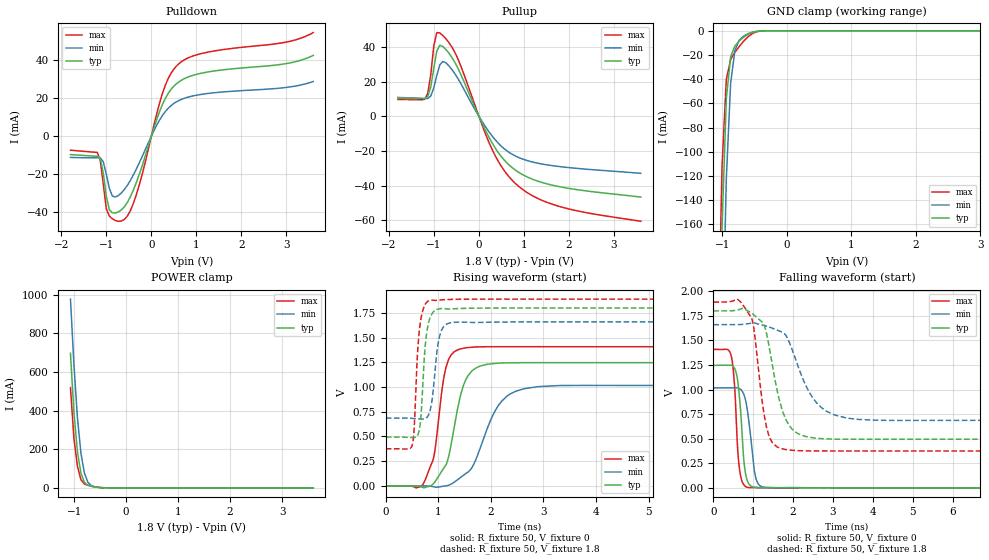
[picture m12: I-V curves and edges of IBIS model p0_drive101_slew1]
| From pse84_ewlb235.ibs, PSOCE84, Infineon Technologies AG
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[Model] p0_drive101_slew1
Model_type I/O
Polarity  Inverting
Enable   Active-High
Vinl  =  0.54
Vinh  =  1.26
Vmeas =  0.9
Cref  =  15pF
| Capacitance   typ   min   max
C_comp   1.253838e-12   1.215159e-12   1.300411e-12
| Variables   typ   min   max
[GND Clamp Reference]   0   0   0
[POWER Clamp Reference]   1.8   1.66   1.89
[Pulldown Reference]   0   0   0
[Pullup Reference]   1.8   1.66   1.89
[Temperature Range]   25   125   -40
[Voltage Range]   1.8   1.66   1.89
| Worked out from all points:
|   slope of the pulldown table from 0 to 0.27 V, typ, clamps not added: 15.1 ohm
|   slope of the pullup table from 0 to 0.27 V, typ, clamps not added: 19 ohm
|   GND clamp passes 1 mA (typ) near -0.51 V on its own axis
|   POWER clamp passes 1 mA (typ) near -0.47 V on its own axis
|   rising waveform, R_fixture 50, V_fixture 0: 20-80 % time 295ps typ, 484ps min, 207ps max; typ from 0 V to 1.25 V
|   rising waveform, R_fixture 50, V_fixture 1.8: 20-80 % time 99.9ps typ, 120ps min, 91.4ps max; typ from 0.495 V to 1.8 V
|   falling waveform, R_fixture 50, V_fixture 0: 20-80 % time 135ps typ, 172ps min, 115ps max; typ from 1.25 V to 0 V
|   falling waveform, R_fixture 50, V_fixture 1.8: 20-80 % time 408ps typ, 637ps min, 275ps max; typ from 1.8 V to 0.495 V
[GND Clamp]
| Voltage   I(typ)   I(min)   I(max)
-1.137V   -619.5mA   -754.2mA   -533mA
-1.07V    -361.2mA   -498.1mA   -281.3mA
-1.003V   -163.8mA   -277.7mA   -113mA
-936.6mV  -56.22mA   -122.3mA   -40.06mA
-869.7mV  -21.33mA   -43.3mA    -23.67mA
-802.8mV  -12.5mA    -15.96mA   -17.71mA
-735.9mV  -8.346mA   -7.675mA   -12.88mA
-669mV    -5.267mA   -4.349mA   -8.575mA
-535.2mV  -1.314mA   -1.207mA   -2.328mA
-401.4mV  -73.55uA   -132.2uA   -119.3uA
3.6V      0A         0A         0A
[POWER Clamp]
| Voltage   I(typ)   I(min)   I(max)
-1.07V    696.7mA    977.2mA    518.8mA
-1.003V   390.1mA    637.2mA    255.1mA
-936.6mV  187.1mA    363.9mA    112.4mA
-869.7mV  77.2mA     180.7mA    42.71mA
-802.8mV  28.89mA    77.43mA    19.98mA
-735.9mV  13.12mA    29.18mA    13.35mA
-669mV    7.754mA    11.55mA    8.954mA
-535.2mV  2.356mA    2.862mA    2.667mA
-334.5mV  34.33uA    127.4uA    15.58uA
3.6V      0A         0A         0A
[Pullup]
| Voltage   I(typ)   I(min)   I(max)
-1.8V     10.42mA    10.91mA    9.748mA
-1.204V   10.14mA    10.34mA    9.878mA
-1.07V    17.03mA    11.78mA    24.18mA
-1.003V   27.73mA    16.47mA    40.58mA
-936.6mV  37.65mA    23.64mA    48.34mA
-869.7mV  41.02mA    29.7mA     48.11mA
-735.9mV  38.62mA    30.93mA    44.83mA
-468.3mV  27.87mA    21.88mA    33.26mA
310.3mV   -16.05mA   -11.89mA   -19.99mA
806.9mV   -30.94mA   -22.81mA   -38.6mA
1.738V    -40.29mA   -28.8mA    -51.57mA
3.6V      -46.58mA   -32.89mA   -60.55mA
[Pulldown]
| Voltage   I(typ)   I(min)   I(max)
-1.8V     -9.752mA   -11.25mA   -7.449mA
-1.204V   -10.63mA   -11.44mA   -8.6mA
-1.137V   -11.77mA   -11.44mA   -12.78mA
-1.003V   -31.53mA   -19.99mA   -38.21mA
-936.6mV  -38.76mA   -27.43mA   -42.02mA
-869.7mV  -40.38mA   -31.49mA   -43.48mA
-669mV    -38.89mA   -29.94mA   -44.72mA
-401.4mV  -28.42mA   -20.48mA   -35.46mA
248.3mV   16.76mA    10.92mA    22.6mA
558.6mV   27.54mA    18.02mA    36.87mA
1.117V    33.09mA    21.95mA    43.43mA
3.6V      42.42mA    28.69mA    54.44mA
[Ramp]
dV/dt_r   0.747895/0.294566n  0.609467/0.484093n  0.845008/0.206684n
dV/dt_f   0.783267/0.408275n  0.583981/0.63745n  0.908802/0.27494n
R_load = 50
[Rising Waveform]
R_fixture = 50
V_fixture = 0
V_fixture_min = 0
V_fixture_max = 0
| Time   V(typ)   V(min)   V(max)
0s        13.05nV    920.4nV    4.73nV
679.4ps   -9.996mV   -46.55uV   -992.9uV
935.9ps   42.41mV    -11.94mV   365.5mV
1.086ns   165.5mV    -4.108mV   1.036V
1.184ns   274.1mV    4.721mV    1.267V
1.432ns   936.3mV    90.17mV    1.388V
1.667ns   1.176V     213mV      1.405V
2.307ns   1.246V     909mV      1.409V
3.307ns   1.247V     1.016V     1.408V
50ns      1.246V     1.016V     1.408V
[Rising Waveform]
R_fixture = 50
V_fixture = 1.8
V_fixture_min = 1.66
V_fixture_max = 1.89
| Time   V(typ)   V(min)   V(max)
0s        494.6mV    686.7mV    375.3mV
502.2ps   488.7mV    683mV      412.8mV
542.1ps   488.9mV    680.8mV    605.7mV
616.6ps   526.3mV    678.2mV    1.45V
664.9ps   684.2mV    676.9mV    1.682V
766.5ps   1.503V     686.6mV    1.852V
861.9ps   1.727V     809.7mV    1.88V
1.036ns   1.793V     1.54V      1.882V
1.358ns   1.794V     1.657V     1.889V
50ns      1.8V       1.66V      1.89V
[Falling Waveform]
R_fixture = 50
V_fixture = 0
V_fixture_min = 0
V_fixture_max = 0
| Time   V(typ)   V(min)   V(max)
0s        1.246V     1.016V     1.408V
424ps     1.249V     1.016V     1.373V
493.6ps   1.237V     1.017V     1.224V
558.6ps   1.191V     1.018V     842.4mV
666.4ps   870.2mV    1.007V     159.1mV
775.3ps   236.4mV    938.5mV    24.99mV
898.1ps   35.95mV    652.6mV    2.836mV
1.071ns   2.872mV    92.03mV    4.303mV
1.383ns   3.767mV    1.785mV    879.7uV
50ns      13.03nV    943.8nV    4.771nV
[Falling Waveform]
R_fixture = 50
V_fixture = 1.8
V_fixture_min = 1.66
V_fixture_max = 1.89
| Time   V(typ)   V(min)   V(max)
0s        1.8V       1.66V      1.89V
598.7ps   1.808V     1.66V      1.919V
962ps     1.777V     1.676V     1.724V
1.251ns   1.674V     1.655V     804mV
1.489ns   1.225V     1.623V     455mV
1.729ns   787.3mV    1.584V     397.5mV
1.926ns   621.1mV    1.46V      383.5mV
2.708ns   500.9mV    817.3mV    375.1mV
4.13ns    494.3mV    687.5mV    375.4mV
50ns      494.6mV    686.7mV    375.3mV
